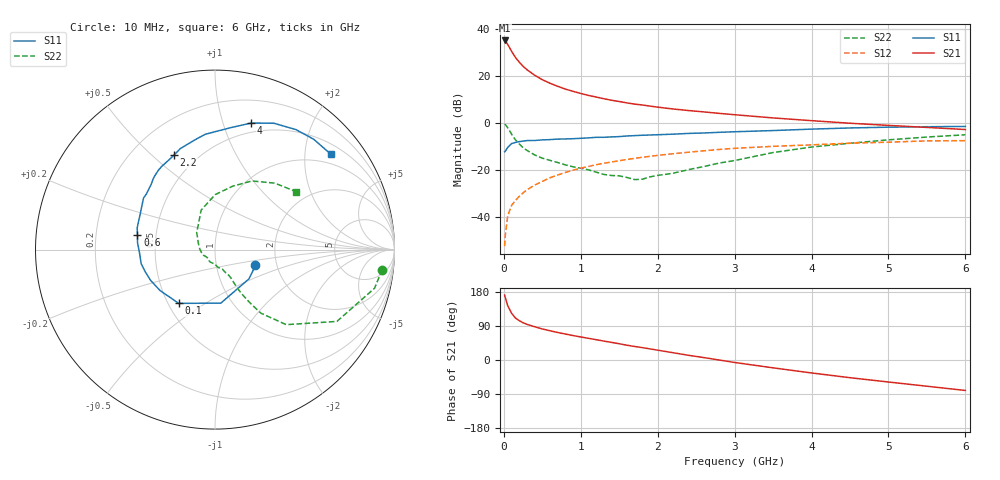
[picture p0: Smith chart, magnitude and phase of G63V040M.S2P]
! SIEMENS Small Signal Semiconductors
! BFG193
! Si NPN RF Bipolar Junction Transistor in SOT223
! VCE = 3 V  IC = 40 mA
! Common Emitter S-Parameters:  August  1996
# GHz  S  MA  R  50
!  f  S11  S21  S12  S22
! GHz  MAG  ANG  MAG  ANG  MAG  ANG  MAG  ANG
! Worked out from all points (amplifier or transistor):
!   36 points, 10 MHz to 6 GHz, reference 50 ohm
!   highest |S21| = 35.0 dB at 10 MHz (marker M1)
!   |S21| within 3 dB of that: start of sweep to 73.12 MHz
!   unconditionally stable (mu >= 1): 462.2 MHz to 2.41 GHz
!   at 250 MHz: K = 0.89, MSG = 26.9 dB, |S12| = -29.8 dB
!   at 1.4 GHz: K = 1.05, MAG = 11.8 dB, |S12| = -16.7 dB
!   at 6 GHz: K = 0.90, MSG = 2.4 dB, |S12| = -7.6 dB
!   S11 on the Smith chart (normalised r, x): 10 MHz: 1.55, -0.29; 100 MHz: 0.57, -0.39; 600 MHz: 0.39, +0.08; 2.2 GHz: 0.38, +0.59; 4 GHz: 0.41, +1.24; 6 GHz: 0.73, +2.60
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0.01  0.242 -21.3  55.97 171.3  0.0024 88.7  0.9381 -6.8
0.02  0.2499 -40.8  54.19 163.9  0.0042 81.3  0.9148 -13.6
0.05  0.3 -83.8  46.19 143.5  0.0105 71.8  0.7884 -30.5
0.1  0.3614 -124.0  33.16 123.6  0.0175 66.6  0.5765 -46.5
0.15  0.3818 -143.3  24.5 111.0  0.0224 64.4  0.4364 -54.2
0.2  0.3979 -154.6  19.39 103.8  0.0273 65.3  0.3554 -56.7
0.25  0.4083 -162.7  15.84 98.3  0.0324 66.1  0.2951 -58.6
0.3  0.4188 -169.1  13.42 94.1  0.0377 67.5  0.2598 -59.6
0.4  0.4208 -177.3  10.23 87.8  0.0474 67.4  0.2081 -60.4
0.5  0.4332 175.0  8.227 81.9  0.0569 66.9  0.1773 -60.8
0.6  0.4392 169.6  6.91 77.2  0.068 66.3  0.1592 -62.1
0.7  0.4501 164.4  5.949 72.6  0.0779 64.8  0.1435 -64.9
0.8  0.4537 160.2  5.197 68.5  0.0883 63.1  0.1277 -67.4
1.1  0.4777 148.1  3.814 57.2  0.1181 58.1  0.1001 -80.5
1.6  0.5247 130.9  2.642 39.0  0.1665 47.3  0.0691 -119.6
2.2  0.5731 113.6  1.963 19.2  0.2206 33.7  0.0848 177.9
2.8  0.6274 98.9  1.584 -0.1  0.2716 19.6  0.1395 137.1
3.5  0.6839 82.9  1.268 -20.7  0.3161 2.4  0.2333 109.3
4  0.7337 74.0  1.109 -34.2  0.3397 -7.4  0.306 89.9
4.5  0.7767 65.0  0.978 -46.7  0.3688 -17.6  0.3674 74.3
5.5  0.8249 48.2  0.797 -69.2  0.413 -40.8  0.4982 48.0
6  0.8358 39.6  0.719 -80.4  0.4176 -54.0  0.5563 35.4
